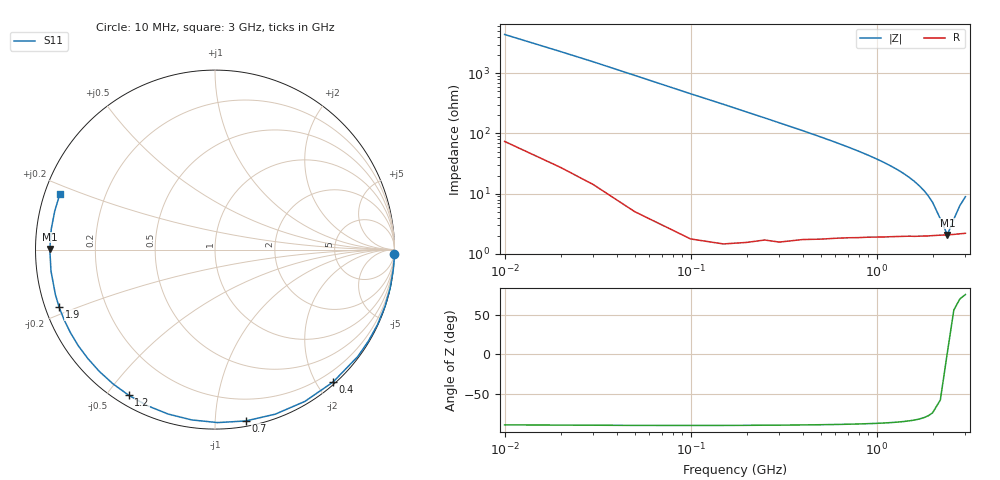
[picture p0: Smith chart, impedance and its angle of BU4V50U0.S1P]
! SIEMENS Small Signal Semiconductors
! BB833
! Si Tuning Diode in SOD323
! VR = 4.5 V
! S-Parameters:  April  1996
# GHz  S  MA  R  50
!  f  S11
! GHz  MAG  ANG
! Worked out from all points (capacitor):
!   31 points, 10 MHz to 3 GHz, reference 50 ohm
!   read as one part to ground: C = 3.47 pF near 10 MHz
!   lowest |Z| = 2.07 ohm at 2.4 GHz (marker M1)
!   series resonance near 2.395 GHz, so ESL is about 1.3 nH
!   S11 on the Smith chart (normalised r, x): 10 MHz: 1, -88; 400 MHz: 0.03, -2.23; 700 MHz: 0.04, -1.20; 1.2 GHz: 0.04, -0.57; 1.9 GHz: 0.04, -0.18; 3 GHz: 0.04, +0.17
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0.01  0.9996 -1.3
0.05  0.9994 -6.2
0.1  0.9992 -12.5
0.15  0.9985 -18.6
0.2  0.9971 -24.8
0.25  0.9952 -30.8
0.3  0.9938 -36.8
0.4  0.9885 -48.3
0.5  0.9829 -59.4
0.6  0.9764 -69.9
0.7  0.9699 -79.8
0.8  0.9639 -89.1
0.9  0.9578 -97.8
1  0.9527 -105.9
1.1  0.9478 -113.5
1.2  0.9433 -120.6
1.3  0.9394 -127.2
1.4  0.9359 -133.5
1.5  0.933 -139.4
1.6  0.9312 -144.9
1.7  0.9289 -150.2
1.9  0.9257 -159.8
2  0.9239 -164.3
2.2  0.9216 -172.6
2.4  0.9204 179.8
2.6  0.9194 172.8
2.8  0.9184 166.4
3  0.918 160.4
